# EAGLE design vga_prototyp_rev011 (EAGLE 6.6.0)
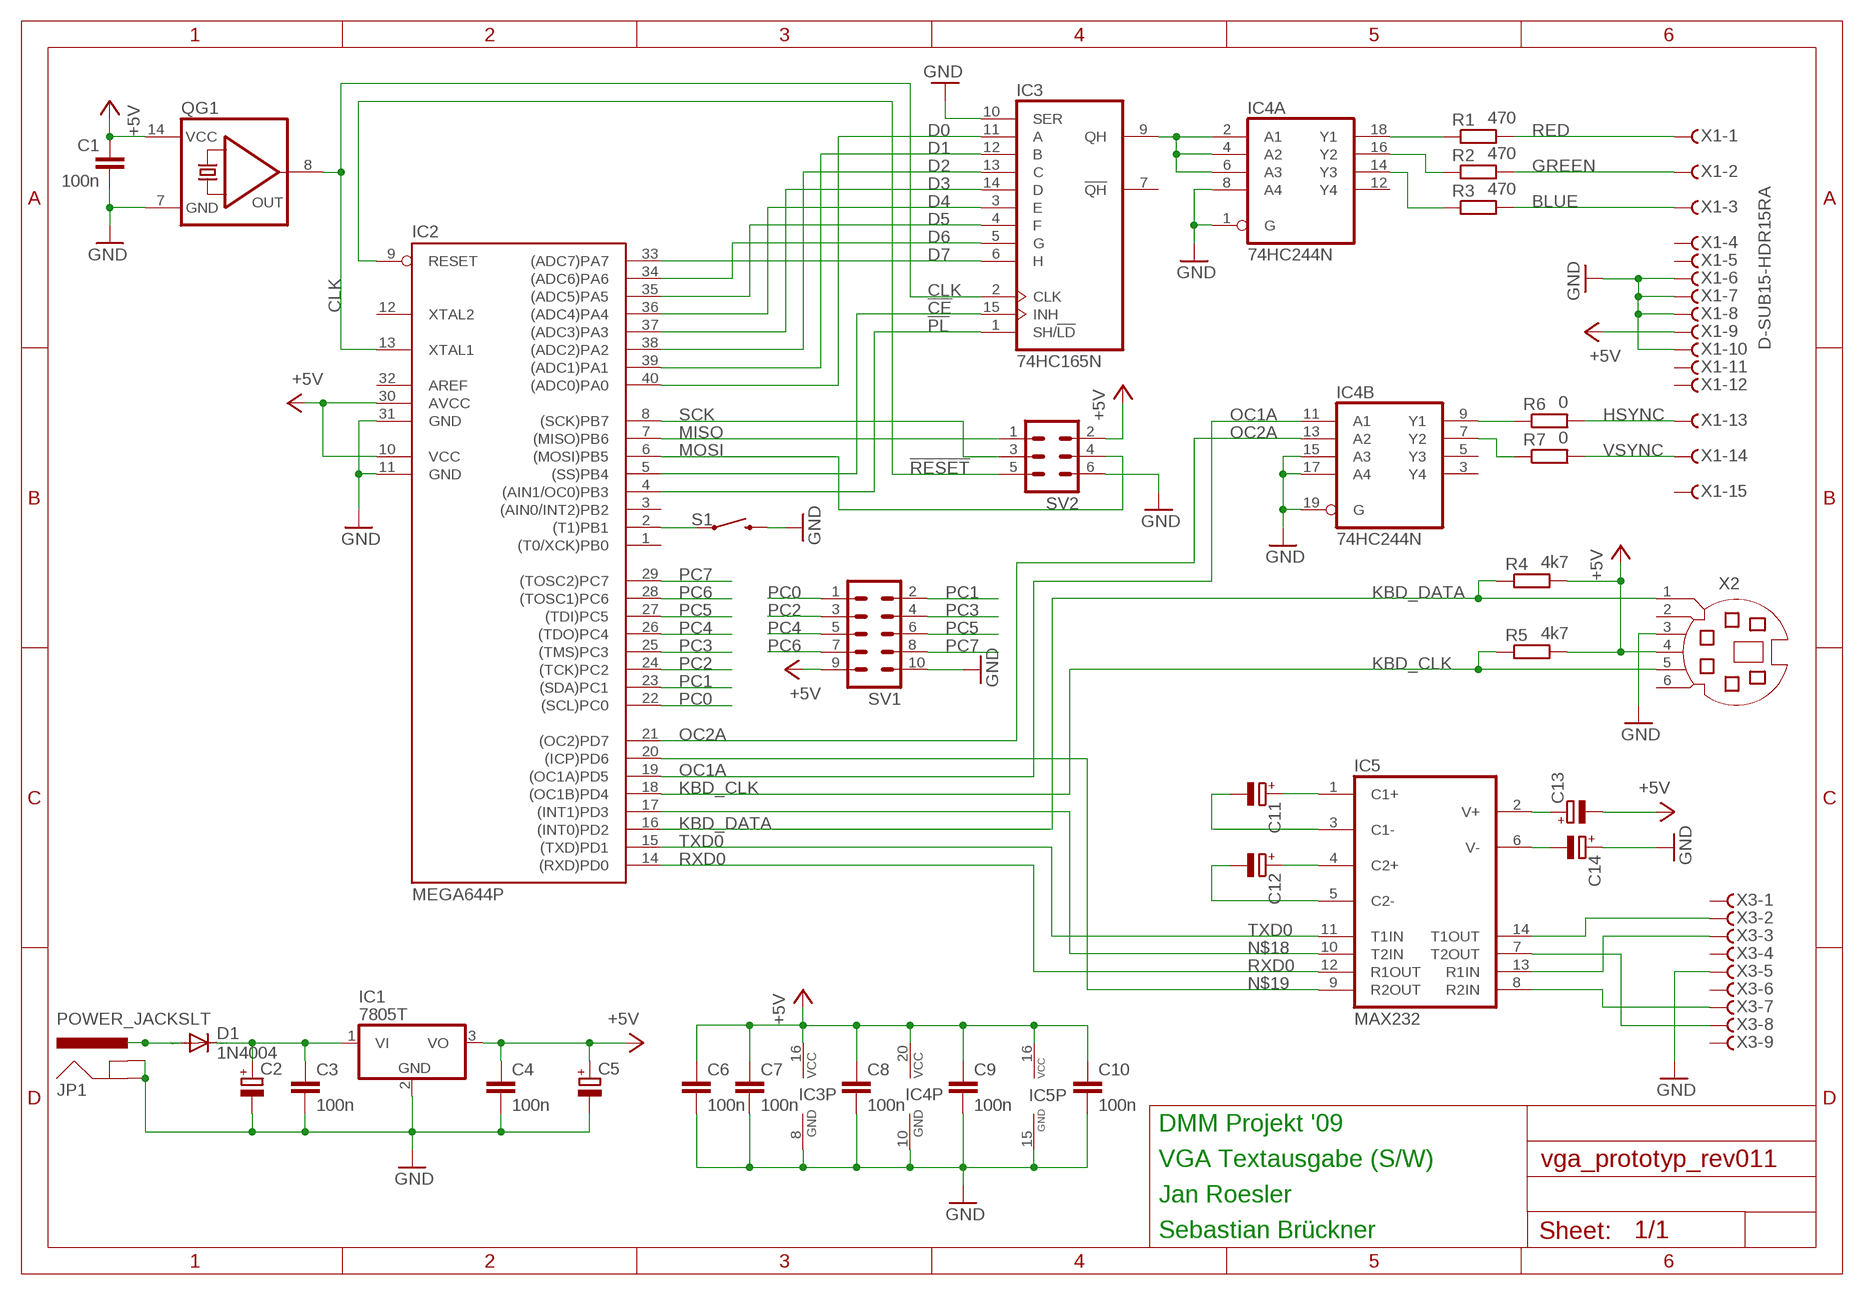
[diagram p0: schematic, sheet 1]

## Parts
C1  100n  C-EU025-025X050  [C025-025X050]
C2  CPOL-EUE5-6  [E5-6]
C3  100n  C-EU025-025X050  [C025-025X050]
C4  100n  C-EU025-025X050  [C025-025X050]
C5  CPOL-EUE5-6  [E5-6]
C6  100n  C-EU025-025X050  [C025-025X050]
C7  100n  C-EU025-025X050  [C025-025X050]
C8  100n  C-EU025-025X050  [C025-025X050]
C9  100n  C-EU025-025X050  [C025-025X050]
C10  100n  C-EU025-025X050  [C025-025X050]
C11  CPOL-EUE2,5-6E  [E2,5-6E]
C12  CPOL-EUE2,5-6E  [E2,5-6E]
C13  CPOL-EUE2,5-6E  [E2,5-6E]
C14  CPOL-EUE2,5-6E  [E2,5-6E]
D1  1N4004  [DO41-10]
IC1  7805T  [TO220H]
IC2  MEGA644P  MEGA16-P  [DIL40]
IC3  74HC165N  [DIL16]
IC4  74HC244N  [DIL20]
IC5  MAX232  [DIL16]
JP1  POWER_JACKSLT  [POWER_JACK_SLOT]
QG1  QG5860  [DIL14S]
R1  470  R-EU_0207/10  [0207/10]
R2  470  R-EU_0207/10  [0207/10]
R3  470  R-EU_0207/10  [0207/10]
R4  4k7  R-EU_0207/10  [0207/10]
R5  4k7  R-EU_0207/10  [0207/10]
R6  0  R-EU_0207/10  [0207/10]
R7  0  R-EU_0207/10  [0207/10]
S1  SWITCH-MOMENTARY-2PTH  [TACTILE-PTH]
SV1  ML10  [ML10]
SV2  ML6  [ML6]
X1  D-SUB15-HDR15RA  [HDR15RA]
X2  MD06SS  [MDIN06SS]
X3  F09HPS  [F09HP]

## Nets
!CE: IC2.5((SS)PB4) IC3.15(INH)
!PL: IC2.4((AIN1/OC0)PB3) IC3.1(SH/!LD)
!RESET: IC2.9(RESET) SV2.5
+5V: C1.1 C4.1 C5.+ C6.1 C7.1 C8.1 C9.1 C10.1 C13.- IC1.3(VO) IC2.10(VCC) IC2.30(AVCC) IC3.16(VCC) IC4.20(P:VCC) IC5.16(VCC) QG1.14(VCC) R4.2 R5.2 SV1.9 SV2.2 X1.9 X2.4
BLUE: R3.2 X1.3
CLK: IC2.13(XTAL1) IC3.2(CLK) QG1.8(OUT)
D0: IC2.40((ADC0)PA0) IC3.11(A)
D1: IC2.39((ADC1)PA1) IC3.12(B)
D2: IC2.38((ADC2)PA2) IC3.13(C)
D3: IC2.37((ADC3)PA3) IC3.14(D)
D4: IC2.36((ADC4)PA4) IC3.3(E)
D5: IC2.35((ADC5)PA5) IC3.4(F)
D6: IC2.34((ADC6)PA6) IC3.5(G)
D7: IC2.33((ADC7)PA7) IC3.6(H)
GND: C1.2 C2.- C3.2 C4.2 C5.- C6.2 C7.2 C8.2 C9.2 C10.2 C14.+ IC1.2(GND) IC2.11(GND) IC2.31(GND) IC3.8(GND) IC3.10(SER) IC4.1(A:G) IC4.8(A:A4) IC4.10(P:GND) IC4.15(B:A3) IC4.17(B:A4) IC4.19(B:G) IC5.15(GND) JP1.GND@1(GNDBREAK) JP1.GND@2(GND) QG1.7(GND) S1.3 SV1.10 SV2.6 X1.6 X1.7 X1.8 X1.10 X2.3 X3.5
GREEN: R2.2 X1.2
HSYNC: R6.2 X1.13
KBD_CLK: IC2.18((OC1B)PD4) R5.1 X2.5
KBD_DATA: IC2.16((INT0)PD2) R4.1 X2.1
MISO: IC2.7((MISO)PB6) SV2.1
MOSI: IC2.6((MOSI)PB5) SV2.4
N$1: IC3.9(QH) IC4.2(A:A1) IC4.4(A:A2) IC4.6(A:A3)
N$2: IC4.18(A:Y1) R1.1
N$3: IC4.16(A:Y2) R2.1
N$4: IC4.14(A:Y3) R3.1
N$5: C2.+ C3.1 D1.C IC1.1(VI)
N$6: C11.+ IC5.1(C1+)
N$7: C11.- IC5.3(C1-)
N$8: C12.+ IC5.4(C2+)
N$9: IC4.9(B:Y1) R6.1
N$10: IC4.7(B:Y2) R7.1
N$11: C12.- IC5.5(C2-)
N$12: C14.- IC5.6(V-)
N$13: C13.+ IC5.2(V+)
N$18: IC2.17((INT1)PD3) IC5.10(T2IN)
N$19: IC2.20((ICP)PD6) IC5.9(R2OUT)
N$20: IC5.14(T1OUT) X3.2
N$21: IC5.13(R1IN) X3.3
N$22: IC5.8(R2IN) X3.7
N$23: IC5.7(T2OUT) X3.8
N$25: IC2.2((T1)PB1) S1.1
OC1A: IC2.19((OC1A)PD5) IC4.11(B:A1)
OC2A: IC2.21((OC2)PD7) IC4.13(B:A2)
PC0: IC2.22((SCL)PC0) SV1.1
PC1: IC2.23((SDA)PC1) SV1.2
PC2: IC2.24((TCK)PC2) SV1.3
PC3: IC2.25((TMS)PC3) SV1.4
PC4: IC2.26((TDO)PC4) SV1.5
PC5: IC2.27((TDI)PC5) SV1.6
PC6: IC2.28((TOSC1)PC6) SV1.7
PC7: IC2.29((TOSC2)PC7) SV1.8
RED: R1.2 X1.1
RXD0: IC2.14((RXD)PD0) IC5.12(R1OUT)
SCK: IC2.8((SCK)PB7) SV2.3
TXD0: IC2.15((TXD)PD1) IC5.11(T1IN)
VSYNC: R7.2 X1.14
X4: D1.A JP1.PWR
Unconnected: IC2.1((T0/XCK)PB0) IC2.3((AIN0/INT2)PB2) IC2.12(XTAL2) IC2.32(AREF) IC3.7(!QH) IC4.3(B:Y4) IC4.5(B:Y3) IC4.12(A:Y4) X1.4 X1.5 X1.11 X1.12 X1.15 X2.2 X2.6 X3.1 X3.4 X3.6 X3.9

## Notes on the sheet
- DMM Projekt '09
- VGA Textausgabe (S/W)
- Jan Roesler
- Sebastian Brückner

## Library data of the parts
C1 C3 C4 C6-C10 = rcl:C-EU: CAPACITOR, European symbol
C2 C5 C11-C14 = rcl:CPOL-EU: POLARIZED CAPACITOR, European symbol
D1 = diode:1N4004: DIODE
IC1 = linear:78*: Positive VOLTAGE REGULATOR Source: http://cache.national.com/ds/LM/LM78L05.pdf http://www.fairchildsemi.com/ds/LM/LM7805.pdf
IC2 = atmel:MEGA16-P: MICROCONTROLLER 16 Kbytes FLASH 1 kbytes SRAM 512 bytes EEPROM USART 8-channel 10 bit ADC Source: avr.lbr
IC3 = 74xx-eu:74*165: 8-bit parallel load SHIFT REGISTER
IC4 = 74xx-eu:74*244: Octal BUFFER and LINE DRIVER, 3-state
IC5 = maxim:MAX232: RS232 TRANSEIVER
JP1 = SparkFun-Connectors:POWER_JACK: Power Jack This is the standard 5.5mm barrel jack for power. The PTH is the most common, proven, reliable, footprint. The Slot footprint only works if the mill layer is transmitted to the PCB fab house so be warned. Mating wall wart : TOL-00298 (and others); PROD_ID: PRT-00119
QG1 = crystal:QG5860: CRYSTAL RESONATOR
R1-R7 = rcl:R-EU_: RESISTOR, European symbol
S1 = SparkFun-Electromechanical:SWITCH-MOMENTARY-2: Various NO switches- pushbuttons, reed, etc; PROD_ID: SWCH-08441
SV1 = con-harting-ml:ML10: HARTING
SV2 = con-harting-ml:ML6: HARTING
X1 = con-thomas-betts:D-SUB15-: D-Subminiatur Connector Source: Electronioc Interconnects European Edition 1998
X2 = con-yamaichi:MD06SS: YAMAICHI CONNECTOR
X3 = con-subd:F09?S: SUB-D

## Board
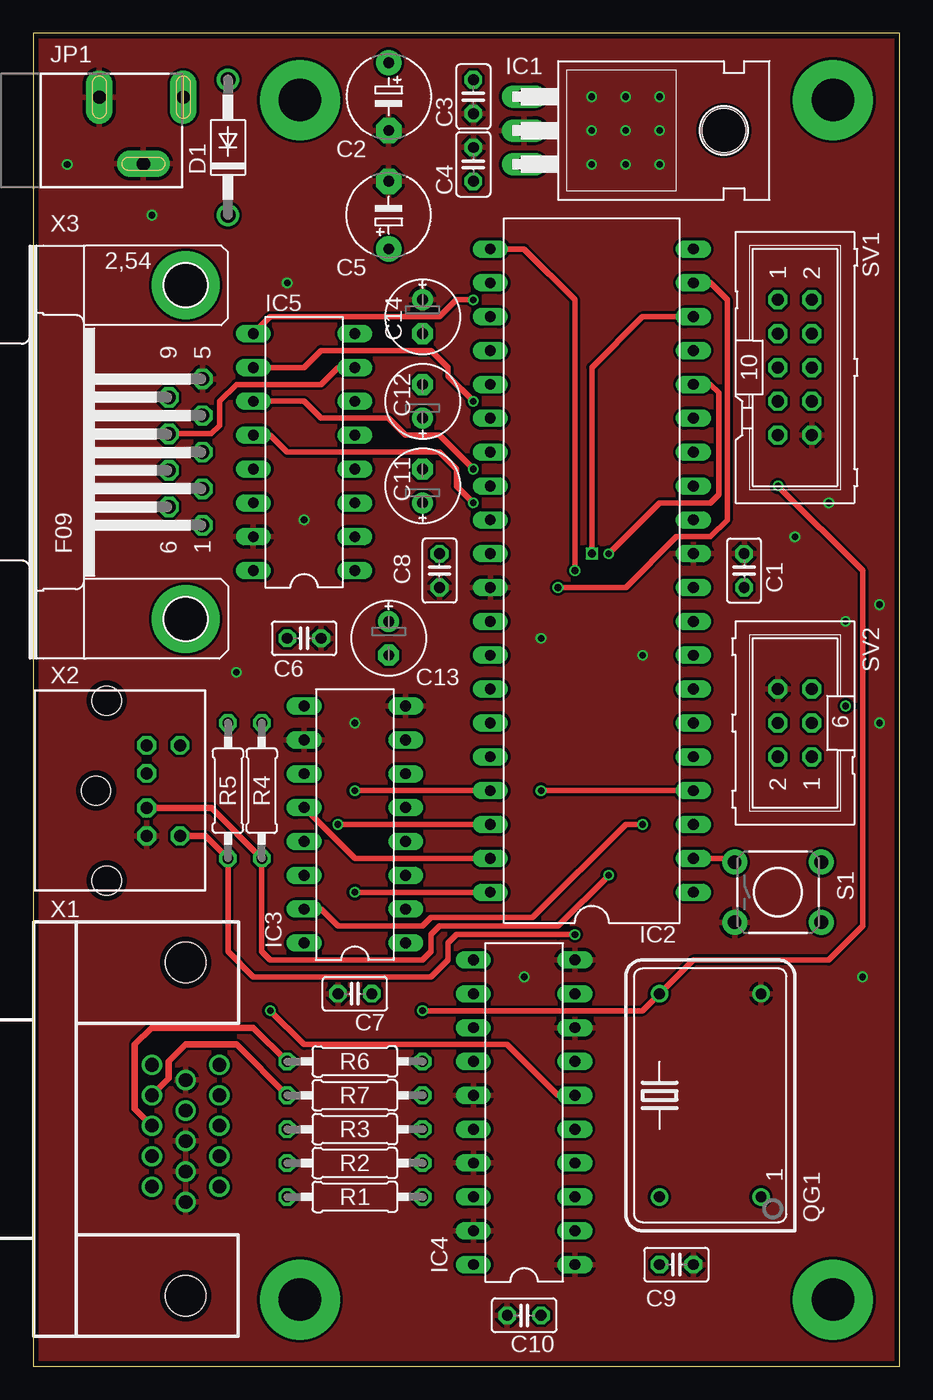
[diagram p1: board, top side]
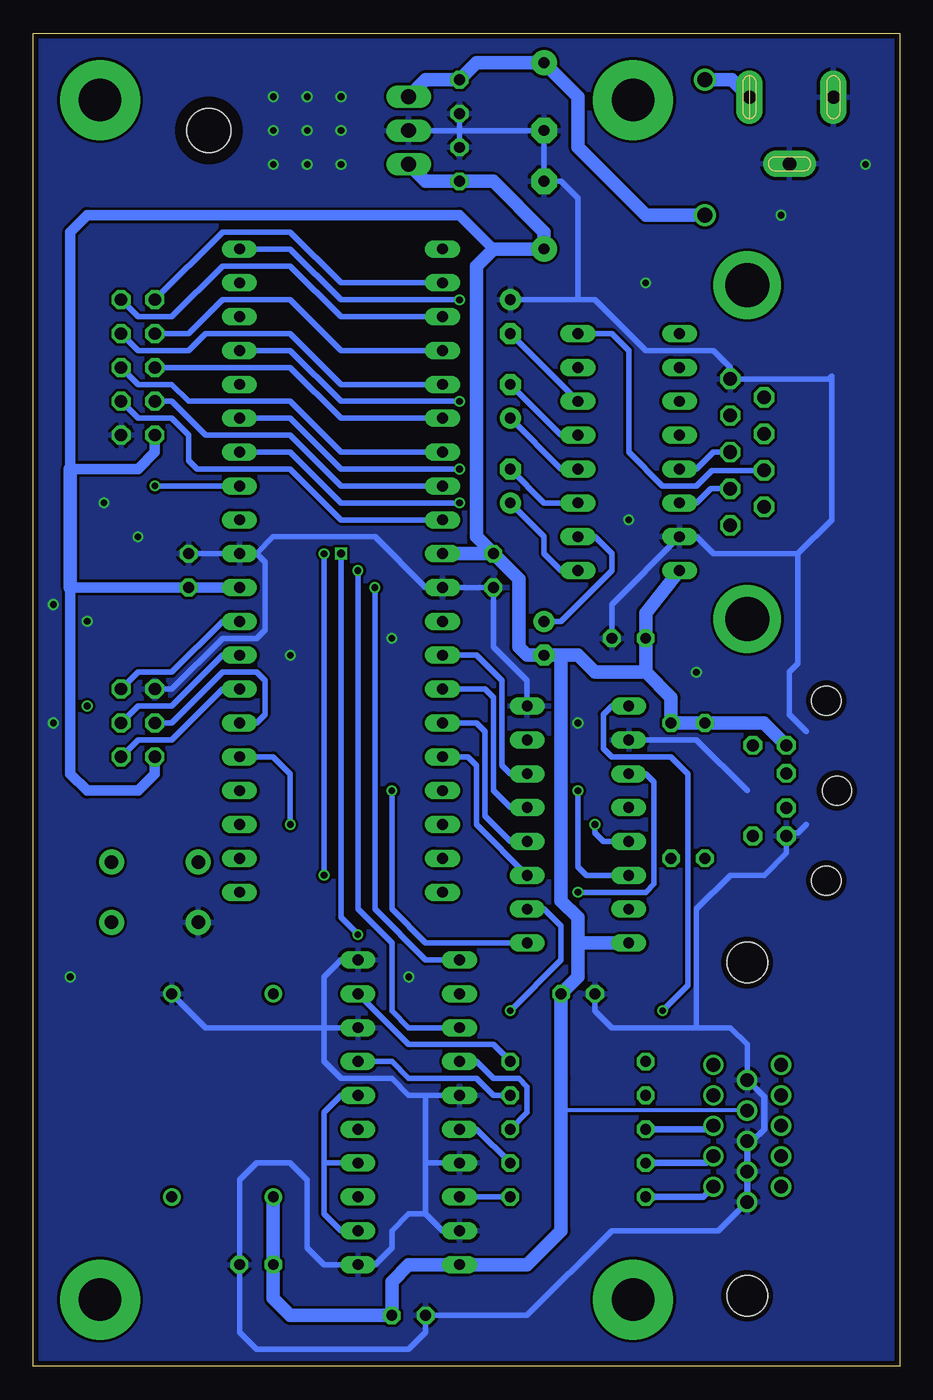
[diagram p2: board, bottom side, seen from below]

Size 65 x 100 mm. Coordinates in mm from the lower left corner, seen from the top.
Outline: 0,0 65,0 65,100 0,100 0,0
Copper layers (1*16): Top 0.035mm / dielectric 1.5mm / Bottom 0.035mm
Design rules "NOA Eagle Rule 2016-06-12 *": minimum track width 6mil, minimum drill 0.3mm, track to track 8mil, track to pad 8mil, pad to pad 8mil, via to via 8mil, smd to smd 0mil, copper to edge 0.4mm, drill to drill 10mil, minimum pad ring 10mil, minimum via ring 6mil, stop-mask expansion 2mil, vias tented up to drill 25mil, thermal gap 10mil

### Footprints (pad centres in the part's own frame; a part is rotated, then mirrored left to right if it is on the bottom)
C025-025X050 = drill 0.813 octagon: 1 -1.27,0; 2 1.27,0
E5-6 = drill 0.813 pad 1.905: + -2.54,0 | drill 0.813 pad 1.905 octagon: - 2.54,0
E2,5-6E = drill 0.813 pad 1.575: + -1.27,0 | drill 0.813 pad 1.575 octagon: - 1.27,0
DO41-10 = drill 1.118: A 5.08,0; C -5.08,0
TO220H = drill 1.118 long: 1 -2.54,-10.16; 2 0,-10.16; 3 2.54,-10.16 | hole 3.302: 0,4.826
DIL40 = drill 0.813 long: 1 -24.13,-7.62; 2 -21.59,-7.62; 3 -19.05,-7.62; 4 -16.51,-7.62; 5 -13.97,-7.62; 6 -11.43,-7.62; 7 -8.89,-7.62; 8 -6.35,-7.62; 9 -3.81,-7.62; 10 -1.27,-7.62; 11 1.27,-7.62; 12 3.81,-7.62; 13 6.35,-7.62; 14 8.89,-7.62; 15 11.43,-7.62; 16 13.97,-7.62; 17 16.51,-7.62; 18 19.05,-7.62; 19 21.59,-7.62; 20 24.13,-7.62; 21 24.13,7.62; 22 21.59,7.62; 23 19.05,7.62; 24 16.51,7.62; 25 13.97,7.62; 26 11.43,7.62; 27 8.89,7.62; 28 6.35,7.62; 29 3.81,7.62; 30 1.27,7.62; 31 -1.27,7.62; 32 -3.81,7.62; 33 -6.35,7.62; 34 -8.89,7.62; 35 -11.43,7.62; 36 -13.97,7.62; 37 -16.51,7.62; 38 -19.05,7.62; 39 -21.59,7.62; 40 -24.13,7.62
DIL16 = drill 0.813 long: 1 -8.89,-3.81; 2 -6.35,-3.81; 3 -3.81,-3.81; 4 -1.27,-3.81; 5 1.27,-3.81; 6 3.81,-3.81; 7 6.35,-3.81; 8 8.89,-3.81; 9 8.89,3.81; 10 6.35,3.81; 11 3.81,3.81; 12 1.27,3.81; 13 -1.27,3.81; 14 -3.81,3.81; 15 -6.35,3.81; 16 -8.89,3.81
DIL20 = drill 0.813 long: 1 -11.43,-3.81; 2 -8.89,-3.81; 3 -6.35,-3.81; 4 -3.81,-3.81; 5 -1.27,-3.81; 6 1.27,-3.81; 7 3.81,-3.81; 8 6.35,-3.81; 9 8.89,-3.81; 10 11.43,-3.81; 11 11.43,3.81; 12 8.89,3.81; 13 6.35,3.81; 14 3.81,3.81; 15 1.27,3.81; 16 -1.27,3.81; 17 -3.81,3.81; 18 -6.35,3.81; 19 -8.89,3.81; 20 -11.43,3.81
POWER_JACK_SLOT = drill 1 pad 2 long: GND@1 2.58,7.5; GND@2 7.58,10.8; PWR 2.58,13.8
DIL14S = drill 0.813: 1 -7.62,-3.81; 7 7.62,-3.81; 8 7.62,3.81; 14 -7.62,3.81
0207/10 = drill 0.813 octagon: 1 -5.08,0; 2 5.08,0
TACTILE-PTH = drill 1.016 pad 1.88: 1 -3.251,2.261; 2 3.251,2.261; 3 -3.251,-2.261; 4 3.251,-2.261
ML10 = drill 0.914 octagon: 1 -5.08,-1.27; 2 -5.08,1.27; 3 -2.54,-1.27; 4 -2.54,1.27; 5 0,-1.27; 6 0,1.27; 7 2.54,-1.27; 8 2.54,1.27; 9 5.08,-1.27; 10 5.08,1.27
ML6 = drill 0.914 octagon: 1 -2.54,-1.27; 2 -2.54,1.27; 3 0,-1.27; 4 0,1.27; 5 2.54,-1.27; 6 2.54,1.27
HDR15RA = drill 1.016: 1 4.318,2.54; 2 2.032,2.54; 3 -0.254,2.54; 4 -2.54,2.54; 5 -4.826,2.54; 6 5.461,0; 7 3.175,0; 8 0.889,0; 9 -1.397,0; 10 -3.683,0; 11 4.318,-2.54; 12 2.032,-2.54; 13 -0.254,-2.54; 14 -2.54,-2.54; 15 -4.826,-2.54 | hole 3.048: -12.497,0; 12.497,0
MDIN06SS = drill 0.9 octagon: 1 1.3,8.5; 2 -1.3,8.5; 3 3.4,8.5; 4 -3.4,8.5; 5 3.4,11; 6 -3.4,11 | hole 2.2: -6.75,5.5; 0,4.7; 6.75,5.5
F09HP = drill 1.016 octagon: 1 -5.486,-1.27; 2 -2.743,-1.27; 3 0,-1.27; 4 2.743,-1.27; 5 5.486,-1.27; 6 -4.115,1.27; 7 -1.372,1.27; 8 1.372,1.27; 9 4.115,1.27 | drill 3.302 pad 5.08: G1 -12.522,0; G2 12.522,0

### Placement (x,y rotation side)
C1  53.34,59.69 90 top
C2  26.67,95.25 270 top
C3  33.02,95.25 270 top
C4  33.02,90.17 90 top
C5  26.67,86.36 90 top
C6  20.32,54.61 0 top
C7  24.13,27.94 180 top
C8  30.48,59.69 270 top
C9  48.26,7.62 0 top
C10  36.83,3.81 180 top
C11  29.21,66.04 90 top
C12  29.21,72.39 90 top
C13  26.67,54.61 270 top
C14  29.21,78.74 270 top
D1  14.61,91.44 90 top
IC1  46.99,92.71 270 top
IC2  41.91,59.69 90 top
IC3  24.13,40.64 90 top
IC4  36.83,19.05 90 top
IC5  20.32,68.58 90 top
JP1  -2.54,97.79 270 top
QG1  50.8,20.32 90 top
R1  24.13,12.7 180 top
R2  24.13,15.24 180 top
R3  24.13,17.78 180 top
R4  17.14,43.18 90 top
R5  14.61,43.18 90 top
R6  24.13,22.86 180 top
R7  24.13,20.32 180 top
S1  55.88,35.56 0 top
SV1  57.15,74.93 270 top
SV2  57.15,48.26 90 top
X1  11.43,17.78 270 top
X2  0,43.18 270 top
X3  11.43,68.58 90 top

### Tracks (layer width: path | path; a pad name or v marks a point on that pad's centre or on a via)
!CE  (via drill 0.5 pad 0.7)
  Top 0.4: IC3.15 21.59,34.29 22.86,33.02 29.21,33.02 29.84,33.66 37.47,33.66 44.45,40.64 v45.72,40.64
  Bottom 0.4: IC2.5 46.99,45.72 45.72,44.45 v45.72,40.64
!PL  (via drill 0.5 pad 0.7)
  Top 0.4: v38.1,43.18 IC2.4
  Bottom 0.4: IC3.1 35.56,31.75 38.1,34.29 v38.1,43.18
!RESET
  Bottom 0.4: SV2.5 57.15,52.07 54.61,52.07 50.8,55.88 IC2.9
+5V
  Bottom 0.3: X1.9 25.53,19.18
  Bottom 0.5: 25.53,19.18 25.4,21.59
  Bottom 0.8: IC2.10 C1.1 62.23,58.42 62.23,44.45 60.96,43.18 57.15,43.18 55.88,44.45 SV2.2 | 30.48,83.82 33.02,86.36 60.96,86.36 62.23,85.09 62.23,67.31 57.15,67.31 55.88,68.58 SV1.9
  Bottom 1: IC1.3 35.56,88.9 C4.1 30.48,88.9 26.67,85.09 C5.+ 30.48,83.82 31.75,82.55 31.75,62.23 C8.1 | C8.1 IC2.30 | C8.1 28.57,59.05 28.57,53.98 27.94,53.34 C13.- 25.4,53.34 | 25.4,53.34 24.13,53.34 22.86,52.07 19.05,52.07 | 19.05,52.07 C6.1 19.05,56.52 IC5.16 | X2.4 10.18,48.26 R5.2 R4.2 17.14,50.16 19.05,52.07 | 24.13,31.75 24.13,29.21 C7.1 25.4,21.59 25.4,10.16 27.94,7.62 IC4.20 36.83,7.62 38.1,6.35 C10.1 45.72,3.81 46.99,5.08 C9.1 QG1.14 | 24.13,31.75 24.13,33.66 25.4,34.92 25.4,53.34 | IC3.16 24.13,31.75 | 62.23,58.42 62.23,67.31
BLUE
  Bottom 0.5: R3.2 14.22,17.78 X1.3
CLK  (via drill 0.5 pad 0.7)
  Top 0.4: v55.88,66.04 62.23,59.69 62.23,33.02 59.69,30.48 49.53,30.48 QG1.8 45.72,26.67 v29.21,26.67
  Bottom 0.4: IC2.13 v55.88,66.04 | IC3.2 26.67,34.29 25.4,33.02 25.4,30.48 v29.21,26.67
D0  (via drill 0.5 pad 0.7)
  Top 0.4: IC2.40 v24.13,35.56
  Bottom 0.4: IC3.11 19.05,44.45 18.41,43.81 18.41,36.2 19.05,35.56 v24.13,35.56
D1
  Top 0.4: IC2.39 24.13,38.1 IC3.12
D2  (via drill 0.5 pad 0.7)
  Top 0.4: IC2.38 v22.86,40.64
  Bottom 0.4: v22.86,40.64 22.86,40.01 22.23,39.37 IC3.13
D3  (via drill 0.5 pad 0.7)
  Top 0.4: IC2.37 v24.13,43.18
  Bottom 0.4: v24.13,43.18 24.13,37.47 23.5,36.83 IC3.14
D4
  Bottom 0.4: IC3.3 31.75,40.64 31.75,45.09 32.38,45.72 IC2.36
D5
  Bottom 0.4: IC3.4 29.21,39.37 31.11,41.27 31.11,47.62 31.75,48.26 IC2.35
D6
  Bottom 0.4: IC3.5 29.21,41.91 30.48,43.18 30.48,50.16 31.11,50.8 IC2.34
D7
  Bottom 0.4: IC3.6 29.21,44.45 29.84,45.09 29.84,51.44 31.75,53.34 IC2.33
GND  (via drill 0.5 pad 0.7)
  Bottom 0.4: IC4.19 34.29,10.16 35.56,11.43 | 35.56,11.43 35.56,15.24 | 35.56,15.24 35.56,20.32 | 35.56,20.32 IC4.15 | IC4.17 35.56,15.24 | 35.56,11.43 36.83,11.43 38.1,10.16 38.1,8.89 39.37,7.62 IC4.1 43.18,7.62 44.45,8.89 44.45,13.97 45.72,15.24 48.26,15.24 49.53,13.97 C9.2 49.53,2.54 48.26,1.27 36.83,1.27 35.56,2.54 C10.2 27.94,3.81 21.59,10.16 13.59,10.16 X1.6 | 35.56,20.32 36.83,20.32 38.1,21.59 41.91,21.59 43.18,22.86 43.18,25.4 | 43.18,25.4 43.18,29.21 41.91,30.48 IC4.10 | IC4.8 43.18,25.4 | QG1.7 52.07,25.4 43.18,25.4 | X1.10 11.43,24.13 12.7,25.4 15.24,25.4 | 15.24,25.4 21.59,25.4 22.86,26.67 C7.2 | 15.24,25.4 15.24,34.29 12.7,36.83 10.16,36.83 8.5,38.49 X2.3 8.28,40.01 7.62,40.01 6.99,40.64 | SV2.6 54.61,50.8 50.8,54.61 48.26,54.61 47.62,55.24 47.62,60.33 48.26,60.96 | 48.26,60.96 IC2.11 C1.2 | IC3.10 15.24,46.99 11.43,43.18 | 48.26,60.96 46.99,62.23 39.37,62.23 35.56,58.42 IC2.31 C8.2 30.48,53.98 27.94,51.44 IC3.8 | 7.62,60.96 5.08,63.5 5.08,74.3 5.31,74.07 X3.5 12.7,74.93 13.97,76.2 19.05,76.2 22.86,80.01 24.13,80.01 | 7.62,60.96 13.97,60.96 15.24,62.23 IC5.15 21.59,57.15 C6.2 | 7.62,60.96 7.62,52.7 8.26,52.07 8.26,48.9 6.99,47.62 | 24.13,80.01 C14.+ | 24.13,80.01 24.13,87.63 25.4,88.9 C5.- C2.- 33.02,92.71 | 33.02,92.71 IC1.2 | C3.2 33.02,92.71 | C4.2 33.02,92.71
  Bottom 0.5: X1.6 X1.7 X1.8 11.05,16.89 10.16,17.78 10.16,20.19 X1.10
  other vias: 63.5,57.15 60.96,55.88 57.15,62.23 59.69,64.77 45.72,53.34 38.1,54.61 41.91,95.25 41.91,92.71 41.91,90.17 44.45,90.17 44.45,92.71 44.45,95.25 46.99,95.25 46.99,92.71 46.99,90.17 63.5,48.26 2.54,90.17 8.89,86.36 19.05,81.28 20.32,63.5 15.24,52.07 24.13,48.26 36.83,29.21 62.23,29.21
  pour Bottom: 0,100 65,100 65,0 0,0
  pour Top: 0,100 65,100 65,0 0,0
GREEN
  Bottom 0.5: X1.2 14.48,15.24 R2.2
HSYNC
  Top 0.5: X1.13 7.62,19.3 7.62,24.13 8.89,25.4 16.51,25.4 R6.2
KBD_CLK  (via drill 0.5 pad 0.7, 0.6)
  Top 0.4: 39.37,32.38 31.75,32.38 31.11,31.75 31.11,30.48 29.84,29.21 16.51,29.21 14.61,31.11 R5.1
  Top 0.406: IC2.18 45.72,78.74 41.91,74.93 v41.91,60.96 | v40.64,32.38 39.37,32.38
  Top 0.5: X2.5 12.93,39.78 R5.1
  Bottom 0.406: v41.91,60.96 41.91,33.66 v40.64,32.38
KBD_DATA  (via drill 0.5 pad 0.7)
  Top 0.4: R4.1 17.14,31.11 17.78,30.48 29.21,30.48 29.84,31.11 29.84,32.38 30.48,33.02 39.37,33.02 v43.18,36.83 | IC2.16 50.8,73.66 51.44,73.03 51.44,65.41 50.8,64.77 46.99,64.77 v43.18,60.96
  Top 0.5: X2.1 13.37,41.88 R4.1
  Bottom 0.4: v43.18,60.96 v43.18,36.83
MISO
  Bottom 0.4: SV2.1 57.15,46.99 54.61,46.99 50.8,50.8 IC2.7
MOSI
  Bottom 0.4: SV2.4 54.61,48.26 50.8,52.07 48.26,52.07 47.62,51.44 47.62,48.9 48.26,48.26 IC2.6
N$1  (via drill 0.5 pad 0.7)
  Top 0.4: IC4.6 39.37,20.32 35.56,24.13 20.32,24.13 v17.78,26.67
  Bottom 0.4: IC4.2 41.91,10.16 43.18,11.43 43.18,15.24 | 43.18,15.24 43.18,19.05 41.91,20.32 IC4.6 | IC4.4 43.18,15.24 | IC3.9 21.59,49.53 22.23,48.9 22.23,46.35 21.59,45.72 17.14,45.72 15.88,44.45 15.88,28.57 v17.78,26.67
N$2
  Bottom 0.4: R1.1 IC4.18
N$3
  Bottom 0.4: IC4.16 31.75,17.78 R2.1
N$4
  Bottom 0.4: IC4.14 31.75,22.86 30.48,21.59 28.57,21.59 27.94,20.95 27.94,19.05 R3.1
N$5
  Bottom 1: IC1.1 35.56,96.52 C3.1 31.75,97.79 C2.+ 24.13,95.25 24.13,91.44 19.05,86.36 D1.C
N$6
  Bottom 0.4: C11.+ 26.67,62.23 26.67,60.96 25.4,59.69 IC5.1
N$7
  Bottom 0.4: C11.- 26.67,64.77 IC5.3
N$8
  Bottom 0.4: C12.+ 25.4,67.31 IC5.4
N$9
  Bottom 0.4: R6.1 30.48,24.13 36.83,24.13 IC4.9
N$10
  Bottom 0.4: R7.1 30.48,20.32 31.75,21.59 36.83,21.59 38.1,22.86 IC4.7
N$11
  Bottom 0.4: C12.- 25.4,69.85 IC5.5
N$12
  Bottom 0.4: C14.- IC5.6
N$13
  Bottom 0.4: IC5.2 22.86,62.23 21.59,60.96 21.59,59.69 25.4,55.88 C13.+
N$15  (via drill 3.2 pad 6)
  other vias: 60,95
N$16  (via drill 3.2 pad 6)
  other vias: 60,5
N$17  (via drill 3.2 pad 6)
  other vias: 20,5
N$18  (via drill 0.5 pad 0.7)
  Top 0.4: IC5.10 20.32,74.93 21.59,76.2 29.84,76.2 31.11,74.93 31.11,74.3 v33.02,72.39
  Bottom 0.4: v33.02,72.39 41.91,72.39 45.72,76.2 IC2.17
N$19  (via drill 0.5 pad 0.7)
  Top 0.4: IC5.9 17.78,78.74 30.48,78.74
  Top 0.406: v33.02,80.01 31.75,80.01 30.48,78.74
  Bottom 0.406: IC2.20 45.72,83.82 41.91,80.01 v33.02,80.01
N$20
  Bottom 0.4: X3.2 14.17,65.84 15.24,64.77 IC5.14
N$21
  Bottom 0.4: X3.3 13.97,68.58 15.24,67.31 IC5.13
N$22
  Bottom 0.4: X3.7 14.07,67.21 15.24,66.04 17.78,66.04 20.32,68.58 20.32,76.2 21.59,77.47 IC5.8
N$23
  Top 0.4: X3.8 13.34,69.95 13.97,70.59 13.97,72.39 15.24,73.66 21.59,73.66 22.86,74.93 IC5.7
N$24  (via drill 3.2 pad 6)
  other vias: 20,95
N$25
  Top 0.4: IC2.2 52.35,38.1 S1.1
N$27  (via drill 0.5 pad 0.7)
  other vias: 60.96,49.53
OC1A  (via drill 0.5 pad 0.7)
  Top 0.4: IC2.19 50.8,81.28 52.07,80.01 52.07,63.5 50.8,62.23 48.26,62.23 44.45,58.42 v39.37,58.42
  Bottom 0.4: IC4.11 35.56,30.48 39.37,34.29 v39.37,58.42
OC2A  (via drill 0.5 pad 0.7)
  Top 0.4: v40.64,59.69 40.64,80.01 36.83,83.82 IC2.21
  Bottom 0.4: IC4.13 36.83,25.4 38.1,26.67 38.1,31.75 40.64,34.29 v40.64,59.69
PC0
  Bottom 0.4: SV1.1 50.8,85.09 45.72,85.09 41.91,81.28 IC2.22
PC1
  Bottom 0.4: SV1.2 57.15,78.74 54.61,78.74 50.8,82.55 45.72,82.55 41.91,78.74 IC2.23
PC2
  Bottom 0.4: SV1.3 53.34,77.47 50.8,80.01 45.72,80.01 41.91,76.2 IC2.24
PC3
  Bottom 0.4: SV1.4 57.15,76.2 53.34,76.2 52.07,77.47 45.72,77.47 41.91,73.66 IC2.25
PC4
  Bottom 0.4: SV1.5 45.72,74.93 41.91,71.12 IC2.26
PC5
  Bottom 0.4: SV1.6 57.15,73.66 54.61,73.66 53.34,72.39 45.72,72.39 41.91,68.58 IC2.27
PC6
  Bottom 0.4: SV1.7 54.61,72.39 52.07,69.85 45.72,69.85 41.91,66.04 IC2.28
PC7
  Bottom 0.4: SV1.8 57.15,71.12 54.61,71.12 53.34,69.85 53.34,67.94 52.7,67.31 45.72,67.31 41.91,63.5 IC2.29
RED
  Bottom 0.5: X1.1 14.73,12.7 R1.2
RXD0  (via drill 0.5 pad 0.7)
  Top 0.4: IC5.12 17.78,69.85 19.05,68.58 30.48,68.58 31.75,67.31 31.75,66.04 v33.02,64.77
  Bottom 0.4: v33.02,64.77 41.91,64.77 45.72,68.58 IC2.14
SCK
  Bottom 0.4: SV2.3 57.15,49.53 54.61,49.53 50.8,53.34 IC2.8
TXD0  (via drill 0.5 pad 0.7)
  Top 0.4: IC5.11 20.32,72.39 21.59,71.12 26.67,71.12 27.94,69.85 30.48,69.85 v33.02,67.31
  Bottom 0.4: v33.02,67.31 41.91,67.31 45.72,71.12 IC2.15
VSYNC
  Top 0.5: X1.14 10.16,21.59 10.16,22.86 11.43,24.13 15.24,24.13 R7.2
X4
  Bottom 1: D1.A 12.57,96.52 JP1.PWR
